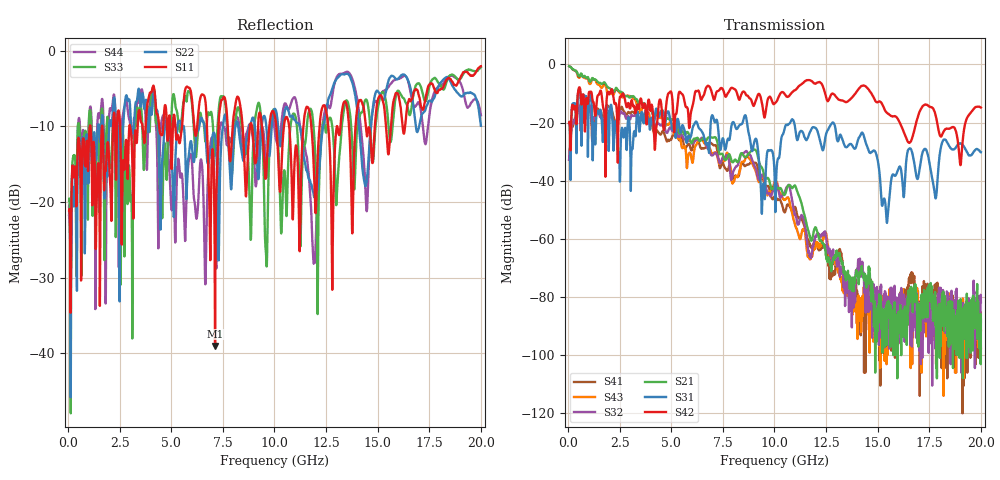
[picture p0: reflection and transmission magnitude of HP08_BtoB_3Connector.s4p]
# MHz S MA R 50.00
! FREQ  S11  S12  S13  S14
!  S21  S22  S23  S24
!  S31  S32  S33  S34
!  S41  S42  S43  S44
!  MAG  ANG  MAG  ANG  MAG  ANG  MAG  ANG
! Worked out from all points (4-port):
!   1996 points, 50 MHz to 20 GHz, reference 50 ohm
!   strongest paths, dB at 50 MHz, 5.04 GHz, 10.03 GHz, 15.02 GHz, 20 GHz:
!     S42: -20.1, -11.1, -13.3, -12.9, -14.8
!     S31: -20.2, -22.1, -46.0, -33.7, -30.2
!     S21: -0.6, -18.9, -41.5, -83.0, -87.7
!     S32: -32.8, -22.8, -41.2, -82.3, -81.7
!     S43: -0.6, -21.4, -40.1, -80.8, -91.4
!     S41: -32.7, -24.9, -45.3, -86.7, -97.7
!   lowest |S11| = -39.0 dB at 7.12 GHz (marker M1), VSWR 1.02, Z = 49 - j0.555 ohm
!   |S11| at or under -10 dB: start of sweep to 1.054 GHz; 6.728 GHz to 7.288 GHz (560 MHz wide, 7.99 % of centre); 10.71 GHz to 11.4 GHz (690.9 MHz wide, 6.25 % of centre)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
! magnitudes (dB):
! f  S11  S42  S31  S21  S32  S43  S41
! 50 MHz  -21.1  -20.1  -20.2  -0.6  -32.8  -0.6  -32.7
! 7.12 GHz  -39.0  -11.3  -19.9  -25.0  -30.4  -30.2  -27.8
! 9.45 GHz  -12.1  -15.8  -41.2  -36.7  -38.2  -38.8  -39.5
! 10.83 GHz  -16.6  -9.8  -19.1  -42.3  -45.8  -50.4  -50.3
! 14.25 GHz  -6.9  -7.3  -23.5  -72.1  -67.9  -79.7  -83.3
! 15.45 GHz  -11.7  -16.7  -54.5  -96.5  -81.9  -98.4  -82.2
! 20 GHz  -2.0  -14.8  -30.2  -87.7  -81.7  -91.4  -97.7
